[IBIS Ver]   3.2
[File name]   apollo7a.ibs
[File Rev]   0.2
[Date]   Mon Oct 28 12:09:41 CST 2002
[Source]   File originated at Motorola Somerset Design Center.
|   Created by Jim Nissen.
[Notes]   This IBIS model is for the Apollo7 483CBGA ceramic package.
|   The driver and receiver models are characterized up to
|   2.5V mode on the data bus and 2.5V mode on the L3
|   interface. The convention is apollox.ibs, where x
|   is one of the configurations of data bus/L3 bus voltage
|   modes. Following is a table of the code for bus combinations:
|   IBIS model   Bus mode   L3 mode
|   apollo7a.ibs   2.5V   2.5V
|   apollo7b.ibs   2.5V   1.8V
|   apollo7c.ibs   2.5V   1.5V
|   apollo7d.ibs   1.8V   2.5V
|   apollo7e.ibs   1.8V   1.8V
|   apollo7f.ibs   1.8V   1.5V
|   apollo7g.ibs   1.5V   2.5V
|   apollo7h.ibs   1.5V   1.8V
|   apollo7i.ibs   1.5V   1.5V
[Disclaimer]   This information is for modeling purposes only and
|   is not guaranteed.
[Component]   Apollo7
[Manufacturer]  Motorola
[Package]
|   typ   min   max
R_pkg   0.0   0.0   0.0
L_pkg   0.0   0.0   0.0
C_pkg   0.0   0.0   0.0
[Pin]   signal_name   model_name  R_pin   L_pin   C_pin
A2   PLL_CFG0   busio   1E-016   1E-016   1E-016
A3   HRESET_   busio   1E-016   1E-016   1E-016
A4   L3VSEL   rcvr   1E-016   1E-016   1E-016
A5   TT3   busio   1E-016   1E-016   1E-016
A6   A8   busio   1E-016   1E-016   1E-016
A7   A6   busio   1E-016   1E-016   1E-016
A9   DX_   busio   1E-016   1E-016   1E-016
A10   A10   busio   1E-016   1E-016   1E-016
A12   L3_DATAP7   l3io   1E-016   1E-016   1E-016
A13   L3_DATA61   l3io   1E-016   1E-016   1E-016
A14   L3_DATA57   l3io   1E-016   1E-016   1E-016
A15   L3_DATAP6   l3io   1E-016   1E-016   1E-016
A16   L3_DATA53   l3io   1E-016   1E-016   1E-016
A17   L3_DATA52   l3io   1E-016   1E-016   1E-016
A18   L3_DATA48   l3io   1E-016   1E-016   1E-016
A19   L3_DATA47   l3io   1E-016   1E-016   1E-016
A20   L3_DATA44   l3io   1E-016   1E-016   1E-016
A21   L3_DATA41   l3io   1E-016   1E-016   1E-016
A22   GND   POWER   1E-016   1E-016   1E-016
B1   GND   POWER   1E-016   1E-016   1E-016
B2   AVDD   POWER   1E-016   1E-016   1E-016
B3   OVDD   POWER   1E-016   1E-016   1E-016
B4   PMON_OUT_   busio   1E-016   1E-016   1E-016
B5   GND   POWER   1E-016   1E-016   1E-016
B6   OSHD_   busio   1E-016   1E-016   1E-016
B7   TBST_   busio   1E-016   1E-016   1E-016
B8   MCP_   busio   1E-016   1E-016   1E-016
B9   EXT_QUAL   busio   1E-016   1E-016   1E-016
B10   CHKS_   busio   1E-016   1E-016   1E-016
B12   GND   POWER   1E-016   1E-016   1E-016
B13   GVDD   POWER   1E-016   1E-016   1E-016
B14   GND   POWER   1E-016   1E-016   1E-016
B15   GVDD   POWER   1E-016   1E-016   1E-016
B16   GND   POWER   1E-016   1E-016   1E-016
B17   GVDD   POWER   1E-016   1E-016   1E-016
B18   GND   POWER   1E-016   1E-016   1E-016
B19   GVDD   POWER   1E-016   1E-016   1E-016
B20   GND   POWER   1E-016   1E-016   1E-016
B21   GVDD   POWER   1E-016   1E-016   1E-016
B22   L3_DATA39   l3io   1E-016   1E-016   1E-016
C1   TRST_   rcvr   1E-016   1E-016   1E-016
C2   PLL_CFG2   busio   1E-016   1E-016   1E-016
C3   GND   POWER   1E-016   1E-016   1E-016
C4   BMODE1_   busio   1E-016   1E-016   1E-016
C5   OVDD   POWER   1E-016   1E-016   1E-016
C6   BMODE0_   busio   1E-016   1E-016   1E-016
C7   OVDD   POWER   1E-016   1E-016   1E-016
C8   A4   busio   1E-016   1E-016   1E-016
C9   GND   POWER   1E-016   1E-016   1E-016
C10   OVDD   POWER   1E-016   1E-016   1E-016
C12   L3_DATA63   l3io   1E-016   1E-016   1E-016
C13   L3_DATA59   l3io   1E-016   1E-016   1E-016
C14   L3_DATA56   l3io   1E-016   1E-016   1E-016
C15   L3_DATA54   l3io   1E-016   1E-016   1E-016
C16   L3_DATA51   l3io   1E-016   1E-016   1E-016
C17   L3_CLK1   l3io   1E-016   1E-016   1E-016
C18   L3_DATA46   l3io   1E-016   1E-016   1E-016
C19   L3_DATA45   l3io   1E-016   1E-016   1E-016
C20   L3_DATAP4   l3io   1E-016   1E-016   1E-016
C21   GND   POWER   1E-016   1E-016   1E-016
C22   L3_DATA36   l3io   1E-016   1E-016   1E-016
D1   TSIZ2   busio   1E-016   1E-016   1E-016
D2   OVDD   POWER   1E-016   1E-016   1E-016
D4   PLL_CFG3   busio   1E-016   1E-016   1E-016
D6   SYSCLK   rcvr   1E-016   1E-016   1E-016
D7   GND   POWER   1E-016   1E-016   1E-016
D8   SRW0_   busio   1E-016   1E-016   1E-016
D9   A35   busio   1E-016   1E-016   1E-016
D10   A32   busio   1E-016   1E-016   1E-016
D12   GVDD   POWER   1E-016   1E-016   1E-016
D13   GND   POWER   1E-016   1E-016   1E-016
D14   GVDD   POWER   1E-016   1E-016   1E-016
D15   GND   POWER   1E-016   1E-016   1E-016
D16   GVDD   POWER   1E-016   1E-016   1E-016
D17   GND   POWER   1E-016   1E-016   1E-016
D18   GVDD   POWER   1E-016   1E-016   1E-016
D19   GND   POWER   1E-016   1E-016   1E-016
D20   L3_DATA38   l3io   1E-016   1E-016   1E-016
D21   GVDD   POWER   1E-016   1E-016   1E-016
D22   L3_DATA33   l3io   1E-016   1E-016   1E-016
E1   TT4   busio   1E-016   1E-016   1E-016
E2   GND   POWER   1E-016   1E-016   1E-016
E3   OVDD   POWER   1E-016   1E-016   1E-016
E4   TDI   rcvr   1E-016   1E-016   1E-016
E05   GND   POWER   1E-016   1E-016   1E-016
E6   PMON_IN_   busio   1E-016   1E-016   1E-016
E8   A2   busio   1E-016   1E-016   1E-016
E9   OVDD   POWER   1E-016   1E-016   1E-016
E10   A0   busio   1E-016   1E-016   1E-016
E12   L3_DATA62   l3io   1E-016   1E-016   1E-016
E13   L3_DATA58   l3io   1E-016   1E-016   1E-016
E14   L3_ECHO_CLK3   l3io   1E-016   1E-016   1E-016
E15   L3_DATA50   l3io   1E-016   1E-016   1E-016
E16   L3_DATAP5   l3io   1E-016   1E-016   1E-016
E17   L3_DATA43   l3io   1E-016   1E-016   1E-016
E18   L3_ECHO_CLK2   l3io   1E-016   1E-016   1E-016
E19   GVDD   POWER   1E-016   1E-016   1E-016
E20   L3_DATA34   l3io   1E-016   1E-016   1E-016
E21   GND   POWER   1E-016   1E-016   1E-016
E22   L3_ADDR15   l3io   1E-016   1E-016   1E-016
F1   TT0   busio   1E-016   1E-016   1E-016
F2   HPR_   busio   1E-016   1E-016   1E-016
F3   CKSTP_IN_   busio   1E-016   1E-016   1E-016
F4   TT1   busio   1E-016   1E-016   1E-016
F5   OVDD   POWER   1E-016   1E-016   1E-016
F6   LSSD_MODE_   rcvr   1E-016   1E-016   1E-016
F7   PLL_CFG1   busio   1E-016   1E-016   1E-016
F8   WAIT_   busio   1E-016   1E-016   1E-016
F9   SRW1_   busio   1E-016   1E-016   1E-016
F10   GND   POWER   1E-016   1E-016   1E-016
F12   GND   POWER   1E-016   1E-016   1E-016
F13   GVDD   POWER   1E-016   1E-016   1E-016
F14   GND   POWER   1E-016   1E-016   1E-016
F15   GVDD   POWER   1E-016   1E-016   1E-016
F16   GND   POWER   1E-016   1E-016   1E-016
F17   GVDD   POWER   1E-016   1E-016   1E-016
F18   L3_DATA37   l3io   1E-016   1E-016   1E-016
F19   GND   POWER   1E-016   1E-016   1E-016
F20   L3_ADDR17   l3io   1E-016   1E-016   1E-016
F21   GVDD   POWER   1E-016   1E-016   1E-016
F22   L3_ADDR12   l3io   1E-016   1E-016   1E-016
G1   SRESET0_   busio   1E-016   1E-016   1E-016
G3   OVDD   POWER   1E-016   1E-016   1E-016
G4   GND   POWER   1E-016   1E-016   1E-016
G5   AP4   busio   1E-016   1E-016   1E-016
G6   BVSEL   rcvr   1E-016   1E-016   1E-016
G7   GND   POWER   1E-016   1E-016   1E-016
G8   SMI0_   busio   1E-016   1E-016   1E-016
G9   OVDD   POWER   1E-016   1E-016   1E-016
G10   A34   busio   1E-016   1E-016   1E-016
G12   L3_DATA60   l3io   1E-016   1E-016   1E-016
G13   L3_DATA55   l3io   1E-016   1E-016   1E-016
G14   L3_DATA49   l3io   1E-016   1E-016   1E-016
G15   L3_DATA42   l3io   1E-016   1E-016   1E-016
G16   L3_DATA40   l3io   1E-016   1E-016   1E-016
G17   GND   POWER   1E-016   1E-016   1E-016
G18   L3_DATA32   l3io   1E-016   1E-016   1E-016
G19   GVDD   POWER   1E-016   1E-016   1E-016
G20   L3_ADDR13   l3io   1E-016   1E-016   1E-016
G21   GND   POWER   1E-016   1E-016   1E-016
G22   L3_ADDR11   l3io   1E-016   1E-016   1E-016
H1   TDO   busio   1E-016   1E-016   1E-016
H2   AP3   busio   1E-016   1E-016   1E-016
H3   TSIZ1   busio   1E-016   1E-016   1E-016
H4   L1_TSTCLK   rcvr   1E-016   1E-016   1E-016
H5   GND   POWER   1E-016   1E-016   1E-016
H6   IARTRY0_   busio   1E-016   1E-016   1E-016
H7   OVDD   POWER   1E-016   1E-016   1E-016
H8   PLL_CFG4   busio   1E-016   1E-016   1E-016
H10   IARTRY1_   busio   1E-016   1E-016   1E-016
H11   L3_ADDR18   l3io   1E-016   1E-016   1E-016
H12   GVDD   POWER   1E-016   1E-016   1E-016
H13   GND   POWER   1E-016   1E-016   1E-016
H14   GVDD   POWER   1E-016   1E-016   1E-016
H15   GND   POWER   1E-016   1E-016   1E-016
H16   L3_DATA35   l3io   1E-016   1E-016   1E-016
H17   GVDD   POWER   1E-016   1E-016   1E-016
H18   L3_ADDR14   l3io   1E-016   1E-016   1E-016
H19   GND   POWER   1E-016   1E-016   1E-016
H20   L3_ADDR10   l3io   1E-016   1E-016   1E-016
H21   GVDD   POWER   1E-016   1E-016   1E-016
H22   L3_ADDR7   l3io   1E-016   1E-016   1E-016
J1   AP2   busio   1E-016   1E-016   1E-016
J2   L2_TSTCLK   busio   1E-016   1E-016   1E-016
J3   GND   POWER   1E-016   1E-016   1E-016
J4   A33   busio   1E-016   1E-016   1E-016
J5   OVDD   POWER   1E-016   1E-016   1E-016
J6   INT0_   busio   1E-016   1E-016   1E-016
J7   TCK   rcvr   1E-016   1E-016   1E-016
J9   VDD   POWER   1E-016   1E-016   1E-016
J10   GND   POWER   1E-016   1E-016   1E-016
J11   VDD   POWER   1E-016   1E-016   1E-016
J12   GND   POWER   1E-016   1E-016   1E-016
J13   VDD   POWER   1E-016   1E-016   1E-016
J14   GND   POWER   1E-016   1E-016   1E-016
J15   VDD   POWER   1E-016   1E-016   1E-016
J16   L3_ADDR16   l3io   1E-016   1E-016   1E-016
J17   GND   POWER   1E-016   1E-016   1E-016
J18   L3_ADDR8   l3io   1E-016   1E-016   1E-016
J19   GVDD   POWER   1E-016   1E-016   1E-016
J20   L3_ADDR6   l3io   1E-016   1E-016   1E-016
J21   GND   POWER   1E-016   1E-016   1E-016
J22   L3_ADDR5   l3io   1E-016   1E-016   1E-016
K1   BR_   busio   1E-016   1E-016   1E-016
K2   HIT_   busio   1E-016   1E-016   1E-016
K3   OVDD   POWER   1E-016   1E-016   1E-016
K4   TMS   rcvr   1E-016   1E-016   1E-016
K5   GND   POWER   1E-016   1E-016   1E-016
K6   CKSTP_OUT_   busio   1E-016   1E-016   1E-016
K7   QACK_   busio   1E-016   1E-016   1E-016
K8   TT2   busio   1E-016   1E-016   1E-016
K9   GND   POWER   1E-016   1E-016   1E-016
K10   VDD   POWER   1E-016   1E-016   1E-016
K11   GND   POWER   1E-016   1E-016   1E-016
K12   VDD   POWER   1E-016   1E-016   1E-016
K13   GND   POWER   1E-016   1E-016   1E-016
K14   VDD   POWER   1E-016   1E-016   1E-016
K15   GND   POWER   1E-016   1E-016   1E-016
K16   L3_ADDR9   l3io   1E-016   1E-016   1E-016
K17   GVDD   POWER   1E-016   1E-016   1E-016
K18   L3_ADDR4   l3io   1E-016   1E-016   1E-016
K19   GND   POWER   1E-016   1E-016   1E-016
K20   L3_ADDR3   l3io   1E-016   1E-016   1E-016
K21   GVDD   POWER   1E-016   1E-016   1E-016
K22   L3_ADDR1   l3io   1E-016   1E-016   1E-016
L1   TSIZ0   busio   1E-016   1E-016   1E-016
L2   WT_   busio   1E-016   1E-016   1E-016
L3   TBEN   busio   1E-016   1E-016   1E-016
L4   SHD0_   busio   1E-016   1E-016   1E-016
L5   AP0   busio   1E-016   1E-016   1E-016
L6   AP1   busio   1E-016   1E-016   1E-016
L7   OVDD   POWER   1E-016   1E-016   1E-016
L8   SHD1_   busio   1E-016   1E-016   1E-016
L9   VDD   POWER   1E-016   1E-016   1E-016
L10   GND   POWER   1E-016   1E-016   1E-016
L11   VDD   POWER   1E-016   1E-016   1E-016
L12   GND   POWER   1E-016   1E-016   1E-016
L13   VDD   POWER   1E-016   1E-016   1E-016
L14   GND   POWER   1E-016   1E-016   1E-016
L15   VDD   POWER   1E-016   1E-016   1E-016
L16   L3_ADDR2   l3io   1E-016   1E-016   1E-016
L17   GND   POWER   1E-016   1E-016   1E-016
L18   L3_ADDR0   l3io   1E-016   1E-016   1E-016
L19   GVDD   POWER   1E-016   1E-016   1E-016
L20   L3_CNTL0   l3io   1E-016   1E-016   1E-016
L21   GND   POWER   1E-016   1E-016   1E-016
L22   L3_CNTL1   l3io   1E-016   1E-016   1E-016
M1   A9   busio   1E-016   1E-016   1E-016
M2   A7   busio   1E-016   1E-016   1E-016
M3   GND   POWER   1E-016   1E-016   1E-016
M4   GBL_   busio   1E-016   1E-016   1E-016
M5   OVDD   POWER   1E-016   1E-016   1E-016
M6   GND   POWER   1E-016   1E-016   1E-016
M7   A23   busio   1E-016   1E-016   1E-016
M8   A14   busio   1E-016   1E-016   1E-016
M9   GND   POWER   1E-016   1E-016   1E-016
M10   VDD   POWER   1E-016   1E-016   1E-016
M11   GND   POWER   1E-016   1E-016   1E-016
M12   VDD   POWER   1E-016   1E-016   1E-016
M13   GND   POWER   1E-016   1E-016   1E-016
M14   VDD   POWER   1E-016   1E-016   1E-016
M15   L3_DATA31   l3io   1E-016   1E-016   1E-016
M16   L3_DATA20   l3io   1E-016   1E-016   1E-016
M17   GVDD   POWER   1E-016   1E-016   1E-016
M18   L3_DATA21   l3io   1E-016   1E-016   1E-016
M19   GND   POWER   1E-016   1E-016   1E-016
M20   L3_DATA22   l3io   1E-016   1E-016   1E-016
M21   GVDD   POWER   1E-016   1E-016   1E-016
M22   L3_DATA23   l3io   1E-016   1E-016   1E-016
N1   CLK_OUT   busio   1E-016   1E-016   1E-016
N2   A12   busio   1E-016   1E-016   1E-016
N3   OVDD   POWER   1E-016   1E-016   1E-016
N4   A1   busio   1E-016   1E-016   1E-016
N5   A3   busio   1E-016   1E-016   1E-016
N6   A16   busio   1E-016   1E-016   1E-016
N7   A24   busio   1E-016   1E-016   1E-016
N8   TA_   busio   1E-016   1E-016   1E-016
N9   VDD   POWER   1E-016   1E-016   1E-016
N10   GND   POWER   1E-016   1E-016   1E-016
N11   VDD   POWER   1E-016   1E-016   1E-016
N12   GND   POWER   1E-016   1E-016   1E-016
N13   VDD   POWER   1E-016   1E-016   1E-016
N14   GND   POWER   1E-016   1E-016   1E-016
N15   VDD   POWER   1E-016   1E-016   1E-016
N16   L3_DATA18   l3io   1E-016   1E-016   1E-016
N17   GND   POWER   1E-016   1E-016   1E-016
N18   L3_DATA16   l3io   1E-016   1E-016   1E-016
N19   GVDD   POWER   1E-016   1E-016   1E-016
N20   L3_DATA17   l3io   1E-016   1E-016   1E-016
N21   GND   POWER   1E-016   1E-016   1E-016
N22   L3_DATA19   l3io   1E-016   1E-016   1E-016
P1   A20   busio   1E-016   1E-016   1E-016
P2   DTI0   busio   1E-016   1E-016   1E-016
P3   GND   POWER   1E-016   1E-016   1E-016
P4   A21   busio   1E-016   1E-016   1E-016
P5   TS_   busio   1E-016   1E-016   1E-016
P6   DTI3   busio   1E-016   1E-016   1E-016
P7   OVDD   POWER   1E-016   1E-016   1E-016
P8   A13   busio   1E-016   1E-016   1E-016
P9   GND   POWER   1E-016   1E-016   1E-016
P10   VDD   POWER   1E-016   1E-016   1E-016
P11   GND   POWER   1E-016   1E-016   1E-016
P12   VDD   POWER   1E-016   1E-016   1E-016
P13   GND   POWER   1E-016   1E-016   1E-016
P14   VDD   POWER   1E-016   1E-016   1E-016
P15   GND   POWER   1E-016   1E-016   1E-016
P16   L3_DATAP3   l3io   1E-016   1E-016   1E-016
P17   GVDD   POWER   1E-016   1E-016   1E-016
P18   L3_DATA29   l3io   1E-016   1E-016   1E-016
P19   GND   POWER   1E-016   1E-016   1E-016
P20   L3_ECHO_CLK1   l3io   1E-016   1E-016   1E-016
P21   GVDD   POWER   1E-016   1E-016   1E-016
P22   L3_DATAP2   l3io   1E-016   1E-016   1E-016
R1   CI_   busio   1E-016   1E-016   1E-016
R2   A5   busio   1E-016   1E-016   1E-016
R3   BG_   busio   1E-016   1E-016   1E-016
R4   OVDD   POWER   1E-016   1E-016   1E-016
R5   A18   busio   1E-016   1E-016   1E-016
R6   A22   busio   1E-016   1E-016   1E-016
R7   D59   busio   1E-016   1E-016   1E-016
R8   DP4   busio   1E-016   1E-016   1E-016
R9   D60   busio   1E-016   1E-016   1E-016
R10   D28   busio   1E-016   1E-016   1E-016
R11   D23   busio   1E-016   1E-016   1E-016
R12   D17   busio   1E-016   1E-016   1E-016
R13   D50   busio   1E-016   1E-016   1E-016
R14   D2   busio   1E-016   1E-016   1E-016
R15   GVDD   POWER   1E-016   1E-016   1E-016
R16   L3_DATA11   l3io   1E-016   1E-016   1E-016
R17   GND   POWER   1E-016   1E-016   1E-016
R18   L3_DATA24   l3io   1E-016   1E-016   1E-016
R19   GVDD   POWER   1E-016   1E-016   1E-016
R20   L3_DATA28   l3io   1E-016   1E-016   1E-016
R21   GND   POWER   1E-016   1E-016   1E-016
R22   L3_DATA30   l3io   1E-016   1E-016   1E-016
T1   TEA_   busio   1E-016   1E-016   1E-016
T2   ARTRY_   busio   1E-016   1E-016   1E-016
T3   OVDD   POWER   1E-016   1E-016   1E-016
T4   GND   POWER   1E-016   1E-016   1E-016
T5   DTI1   busio   1E-016   1E-016   1E-016
T6   DRDY_   busio   1E-016   1E-016   1E-016
T7   GND   POWER   1E-016   1E-016   1E-016
T8   D33   busio   1E-016   1E-016   1E-016
T9   GND   POWER   1E-016   1E-016   1E-016
T10   D25   busio   1E-016   1E-016   1E-016
T11   D22   busio   1E-016   1E-016   1E-016
T12   D14   busio   1E-016   1E-016   1E-016
T13   GND   POWER   1E-016   1E-016   1E-016
T14   D1   busio   1E-016   1E-016   1E-016
T15   GND   POWER   1E-016   1E-016   1E-016
T16   L3_DATA7   l3io   1E-016   1E-016   1E-016
T17   GVDD   POWER   1E-016   1E-016   1E-016
T18   L3_DATA14   l3io   1E-016   1E-016   1E-016
T19   GND   POWER   1E-016   1E-016   1E-016
T20   L3_DATA25   l3io   1E-016   1E-016   1E-016
T21   GVDD   POWER   1E-016   1E-016   1E-016
T22   L3_DATA27   l3io   1E-016   1E-016   1E-016
U1   AACK_   busio   1E-016   1E-016   1E-016
U2   A11   busio   1E-016   1E-016   1E-016
U3   DTI2   busio   1E-016   1E-016   1E-016
U4   A26   busio   1E-016   1E-016   1E-016
U5   OVDD   POWER   1E-016   1E-016   1E-016
U6   A17   busio   1E-016   1E-016   1E-016
U7   OVDD   POWER   1E-016   1E-016   1E-016
U8   DP6   busio   1E-016   1E-016   1E-016
U9   D31   busio   1E-016   1E-016   1E-016
U10   D29   busio   1E-016   1E-016   1E-016
U11   OVDD   POWER   1E-016   1E-016   1E-016
U12   D10   busio   1E-016   1E-016   1E-016
U13   D13   busio   1E-016   1E-016   1E-016
U14   D5   busio   1E-016   1E-016   1E-016
U15   OVDD   POWER   1E-016   1E-016   1E-016
U16   L3_DATA2   l3io   1E-016   1E-016   1E-016
U17   GND   POWER   1E-016   1E-016   1E-016
U18   L3_DATA9   l3io   1E-016   1E-016   1E-016
U19   GVDD   POWER   1E-016   1E-016   1E-016
U20   L3_DATA15   l3io   1E-016   1E-016   1E-016
U21   GND   POWER   1E-016   1E-016   1E-016
U22   L3_DATA26   l3io   1E-016   1E-016   1E-016
V1   DBG_   busio   1E-016   1E-016   1E-016
V2   GND   POWER   1E-016   1E-016   1E-016
V3   OVDD   POWER   1E-016   1E-016   1E-016
V4   A30   busio   1E-016   1E-016   1E-016
V5   GND   POWER   1E-016   1E-016   1E-016
V6   D56   busio   1E-016   1E-016   1E-016
V7   D32   busio   1E-016   1E-016   1E-016
V8   GND   POWER   1E-016   1E-016   1E-016
V9   OVDD   POWER   1E-016   1E-016   1E-016
V10   D27   busio   1E-016   1E-016   1E-016
V11   D21   busio   1E-016   1E-016   1E-016
V12   GND   POWER   1E-016   1E-016   1E-016
V13   OVDD   POWER   1E-016   1E-016   1E-016
V14   D4   busio   1E-016   1E-016   1E-016
V15   GND   POWER   1E-016   1E-016   1E-016
V16   D53   busio   1E-016   1E-016   1E-016
V17   GVDD   POWER   1E-016   1E-016   1E-016
V18   L3_ECHO_CLK0   l3io   1E-016   1E-016   1E-016
V19   GND   POWER   1E-016   1E-016   1E-016
V20   L3_DATA12   l3io   1E-016   1E-016   1E-016
V21   GVDD   POWER   1E-016   1E-016   1E-016
V22   L3_CLK0   l3io   1E-016   1E-016   1E-016
W1   A28   busio   1E-016   1E-016   1E-016
W2   A27   busio   1E-016   1E-016   1E-016
W3   A29   busio   1E-016   1E-016   1E-016
W4   A15   busio   1E-016   1E-016   1E-016
W5   DP5   busio   1E-016   1E-016   1E-016
W6   D54   busio   1E-016   1E-016   1E-016
W7   GND   POWER   1E-016   1E-016   1E-016
W8   D40   busio   1E-016   1E-016   1E-016
W9   D63   busio   1E-016   1E-016   1E-016
W10   D24   busio   1E-016   1E-016   1E-016
W11   D26   busio   1E-016   1E-016   1E-016
W12   D15   busio   1E-016   1E-016   1E-016
W13   D11   busio   1E-016   1E-016   1E-016
W14   D49   busio   1E-016   1E-016   1E-016
W15   D51   busio   1E-016   1E-016   1E-016
W16   D7   busio   1E-016   1E-016   1E-016
W17   GND   POWER   1E-016   1E-016   1E-016
W18   L3_DATA3   l3io   1E-016   1E-016   1E-016
W19   GVDD   POWER   1E-016   1E-016   1E-016
W20   L3_DATA8   l3io   1E-016   1E-016   1E-016
W21   GND   POWER   1E-016   1E-016   1E-016
W22   L3_DATA13   l3io   1E-016   1E-016   1E-016
Y1   QREQ_   busio   1E-016   1E-016   1E-016
Y2   OVDD   POWER   1E-016   1E-016   1E-016
Y3   GND   POWER   1E-016   1E-016   1E-016
Y4   A19   busio   1E-016   1E-016   1E-016
Y5   OVDD   POWER   1E-016   1E-016   1E-016
Y6   D35   busio   1E-016   1E-016   1E-016
Y7   OVDD   POWER   1E-016   1E-016   1E-016
Y8   D38   busio   1E-016   1E-016   1E-016
Y9   GND   POWER   1E-016   1E-016   1E-016
Y10   OVDD   POWER   1E-016   1E-016   1E-016
Y11   D9   busio   1E-016   1E-016   1E-016
Y12   D20   busio   1E-016   1E-016   1E-016
Y13   GND   POWER   1E-016   1E-016   1E-016
Y14   D12   busio   1E-016   1E-016   1E-016
Y15   GND   POWER   1E-016   1E-016   1E-016
Y16   D47   busio   1E-016   1E-016   1E-016
Y17   OVDD   POWER   1E-016   1E-016   1E-016
Y18   D45   busio   1E-016   1E-016   1E-016
Y19   OVDD   POWER   1E-016   1E-016   1E-016
Y20   GND   POWER   1E-016   1E-016   1E-016
Y21   GVDD   POWER   1E-016   1E-016   1E-016
Y22   L3_DATA10   l3io   1E-016   1E-016   1E-016
AA1   A31   busio   1E-016   1E-016   1E-016
AA2   DP0   busio   1E-016   1E-016   1E-016
AA3   A25   busio   1E-016   1E-016   1E-016
AA4   OVDD   POWER   1E-016   1E-016   1E-016
AA5   GND   POWER   1E-016   1E-016   1E-016
AA6   D37   busio   1E-016   1E-016   1E-016
AA7   D39   busio   1E-016   1E-016   1E-016
AA8   DP3   busio   1E-016   1E-016   1E-016
AA9   D61   busio   1E-016   1E-016   1E-016
AA10   D30   busio   1E-016   1E-016   1E-016
AA11   D8   busio   1E-016   1E-016   1E-016
AA12   D55   busio   1E-016   1E-016   1E-016
AA13   D18   busio   1E-016   1E-016   1E-016
AA14   D52   busio   1E-016   1E-016   1E-016
AA15   OVDD   POWER   1E-016   1E-016   1E-016
AA16   D42   busio   1E-016   1E-016   1E-016
AA17   GND   POWER   1E-016   1E-016   1E-016
AA18   D48   busio   1E-016   1E-016   1E-016
AA19   L3_DATA0   l3io   1E-016   1E-016   1E-016
AA20   L3_DATA4   l3io   1E-016   1E-016   1E-016
AA21   L3_DATA6   l3io   1E-016   1E-016   1E-016
AA22   L3_DATAP1   l3io   1E-016   1E-016   1E-016
AB1   GND   POWER   1E-016   1E-016   1E-016
AB2   DP2   busio   1E-016   1E-016   1E-016
AB3   DP1   busio   1E-016   1E-016   1E-016
AB4   D34   busio   1E-016   1E-016   1E-016
AB5   DP7   busio   1E-016   1E-016   1E-016
AB6   D58   busio   1E-016   1E-016   1E-016
AB7   D36   busio   1E-016   1E-016   1E-016
AB8   D62   busio   1E-016   1E-016   1E-016
AB9   D57   busio   1E-016   1E-016   1E-016
AB10   D41   busio   1E-016   1E-016   1E-016
AB11   D19   busio   1E-016   1E-016   1E-016
AB12   D16   busio   1E-016   1E-016   1E-016
AB13   D3   busio   1E-016   1E-016   1E-016
AB14   D6   busio   1E-016   1E-016   1E-016
AB15   D0   busio   1E-016   1E-016   1E-016
AB16   D43   busio   1E-016   1E-016   1E-016
AB17   D44   busio   1E-016   1E-016   1E-016
AB18   D46   busio   1E-016   1E-016   1E-016
AB19   L3_DATAP0   l3io   1E-016   1E-016   1E-016
AB20   L3_DATA1   l3io   1E-016   1E-016   1E-016
AB21   L3_DATA5   l3io   1E-016   1E-016   1E-016
AB22   GND   POWER   1E-016   1E-016   1E-016
|!!!![Package Model] 'name'  calls name
[Package Model] apollo7_483
[Define Package Model] apollo7_483
[Manufacturer] Motorola Inc.
[OEM] Motorola Inc.
[Description] Apollo7 483 CBGA Package T-Line pkg model
[Number Of Sections] 29
[Number Of Pins]  281
[Pin Numbers]
|Although any length unit can be used for Len, mm is used here.
|signal (1)A(10)
A10   Len=0 L=0.0115888305n /
Len=0 L=0.0115888305n /
Len=0 L=0.0115888305n /
Len=0 L=0.0115888305n /
Len=0 L=0.0115888305n /
Len=13.41889 L=0.40648702n C=0.28033364p R=0.015902141 /
Len=0 L=0.0115888305n /
Len=0 L=0.0115888305n /
Len=0 L=0.0115888305n /
Len=0 L=0.027n /
|signal (2)L3_DATAP(7)
A12   Len=0 L=0.0115888305n /
Len=0 L=0.0115888305n /
Len=0 L=0.0115888305n /
Len=11.64898 L=0.3948527n C=0.28900883p R=0.014814815 /
Len=0 L=0.0115888305n /
Len=3.85077 L=0.3948527n C=0.28900883p R=0.014814815 /
Len=0 L=0.0115888305n /
Len=4.88358 L=0.3948527n C=0.28900883p R=0.014814815 /
Len=0 L=0.0115888305n /
Len=0 L=0.0115888305n /
Len=0 L=0.0115888305n /
Len=0 L=0.0115888305n /
Len=0 L=0.0115888305n /
Len=0 L=0.027n /
|signal (3)L3_DATA(61)
A13   Len=0 L=0.0115888305n /
Len=0 L=0.0115888305n /
Len=0 L=0.0115888305n /
Len=9.55053 L=0.3948527n C=0.28900883p R=0.014814815 /
Len=0 L=0.0115888305n /
Len=0 L=0.0115888305n /
Len=0 L=0.0115888305n /
Len=0 L=0.0115888305n /
Len=0.706 L=0.50999594n C=0.25353685p R=0.017094018 /
Len=0 L=0.0115888305n /
Len=0 L=0.0115888305n /
Len=2.03641 L=0.3948527n C=0.28900883p R=0.014814815 /
Len=0 L=0.0115888305n /
Len=0 L=0.0115888305n /
Len=2.259 L=0.50999594n C=0.25353685p R=0.017094018 /
Len=0 L=0.0115888305n /
Len=0 L=0.0115888305n /
Len=0 L=0.0115888305n /
Len=0 L=0.0115888305n /
Len=5.8358  L=0.3948527n C=0.28900883p R=0.014814815 /
Len=0 L=0.0115888305n /
Len=0 L=0.0115888305n /
Len=0 L=0.0115888305n /
Len=0 L=0.0115888305n /
Len=0 L=0.0115888305n /
Len=0 L=0.027n /
|signal (4)L3_DATA(57)
A14   Len=0 L=0.0115888305n /
Len=0 L=0.0115888305n /
Len=0 L=0.0115888305n /
Len=1.8156348 L=0.3948527n C=0.28900883p R=0.014814815 /
Len=0 L=0.0115888305n /
Len=0 L=0.0115888305n /
Len=0.7243503 L=0.3948527n C=0.28900883p R=0.014814815 /
Len=0 L=0.0115888305n /
Len=0 L=0.0115888305n /
Len=17.844217 L=0.50999594n C=0.25353685p R=0.017094018 /
Len=0 L=0.0115888305n /
Len=0 L=0.027n /
|signal (5)L3_DATAP(6)
A15   Len=0 L=0.0115888305n /
Len=0 L=0.0115888305n /
Len=0 L=0.0115888305n /
Len=12.739074 L=0.41058078n C=0.27740377p R=0.016306954 /
Len=0 L=0.0115888305n /
Len=0 L=0.0115888305n /
Len=3.2260232 L=0.3948527n C=0.28900883p R=0.014814815 /
Len=0 L=0.0115888305n /
Len=0 L=0.0115888305n /
Len=4.40548 L=0.4856581n C=0.26624238p R=0.014814815 /
Len=0 L=0.0115888305n /
Len=0 L=0.027n /
|signal (6)L3_DATA(53)
A16   Len=0 L=0.0115888305n /
Len=0 L=0.0115888305n /
Len=0 L=0.0115888305n /
Len=0 L=0.0115888305n /
Len=0 L=0.0115888305n /
Len=0 L=0.0115888305n /
Len=0 L=0.0115888305n /
Len=20.398748 L=0.49811226n C=0.25958562p R=0.015932914 /
Len=0 L=0.0115888305n /
Len=0 L=0.027n /
|signal (7)L3_DATA(52)
A17   Len=0 L=0.0115888305n /
Len=0 L=0.0115888305n /
Len=0 L=0.0115888305n /
Len=0 L=0.0115888305n /
Len=0 L=0.0115888305n /
Len=12.036658 L=0.42205358n C=0.26950994p R=0.017508417 /
Len=0 L=0.0115888305n /
Len=0 L=0.0115888305n /
Len=8.099174 L=0.4856581n C=0.26624238p R=0.014814815 /
Len=0 L=0.0115888305n /
Len=0 L=0.027n /
|signal (8)L3_DATA(48)
A18   Len=0 L=0.0115888305n /
Len=0 L=0.0115888305n /
Len=0 L=0.0115888305n /
Len=20.387503 L=0.3979373n C=0.2866569p R=0.015094339 /
Len=0 L=0.0115888305n /
Len=0 L=0.0115888305n /
Len=0 L=0.0115888305n /
Len=0 L=0.0115888305n /
Len=0 L=0.0115888305n /
Len=0 L=0.027n /
|signal (9)L3_DATA(47)
A19   Len=0 L=0.0115888305n /
Len=0 L=0.0115888305n /
Len=0 L=0.0115888305n /
Len=6.161309 L=0.3948527n C=0.28900883p R=0.014814815 /
Len=0 L=0.0115888305n /
Len=0 L=0.0115888305n /
Len=7.244859 L=0.3948527n C=0.28900883p R=0.014814815 /
Len=0 L=0.0115888305n /
Len=0 L=0.0115888305n /
Len=6.841765 L=0.51434404n C=0.25139356p R=0.01754386 /
Len=0 L=0.0115888305n /
Len=0 L=0.027n /
|signal (10)PLL_CFG(0)
A2   Len=0 L=0.0115888305n /
Len=0 L=0.0115888305n /
Len=0 L=0.0115888305n /
Len=17.249193 L=0.40563312n C=0.2809526p R=0.015819209 /
Len=0 L=0.0115888305n /
Len=0 L=0.0115888305n /
Len=0 L=0.0115888305n /
Len=0 L=0.0115888305n /
Len=0 L=0.0115888305n /
Len=0 L=0.027n /
|signal (11)L3_DATA(44)
A20   Len=0 L=0.0115888305n /
Len=0 L=0.0115888305n /
Len=0 L=0.0115888305n /
Len=0 L=0.0115888305n /
Len=0 L=0.0115888305n /
Len=9.950993 L=0.40513027n C=0.2813184p R=0.015770609 /
Len=0 L=0.0115888305n /
Len=0 L=0.0115888305n /
Len=10.417507 L=0.4856581n C=0.26624238p R=0.014814815 /
Len=0 L=0.0115888305n /
Len=0 L=0.027n /
|signal (12)L3_DATA(41)
A21   Len=0 L=0.0115888305n /
Len=0 L=0.0115888305n /
Len=0 L=0.0115888305n /
Len=0 L=0.0115888305n /
Len=0 L=0.0115888305n /
Len=10.842759 L=0.3948527n C=0.28900883p R=0.014814815 /
Len=0 L=0.0115888305n /
Len=0 L=0.0115888305n /
Len=9.295238 L=0.51288456n C=0.25210893p R=0.017391305 /
Len=0 L=0.0115888305n /
Len=0 L=0.027n /
|signal (13)HRESET_B
A3   Len=0 L=0.0115888305n /
Len=0 L=0.0115888305n /
Len=0 L=0.0115888305n /
Len=16.309668 L=0.4141186n C=0.27492067p R=0.016666668 /
Len=0 L=0.0115888305n /
Len=0 L=0.0115888305n /
Len=0 L=0.0115888305n /
Len=0 L=0.0115888305n /
Len=0 L=0.0115888305n /
Len=0 L=0.027n /
|signal (14)L3VSEL
A4   Len=0 L=0.0115888305n /
Len=0 L=0.0115888305n /
Len=0 L=0.0115888305n /
Len=9.143236 L=0.40563312n C=0.2809526p R=0.015819209 /
Len=0 L=0.0115888305n /
Len=0 L=0.0115888305n /
Len=0 L=0.0115888305n /
Len=0 L=0.0115888305n /
Len=8.76985 L=0.4856581n C=0.26624238p R=0.014814815 /
Len=0 L=0.0115888305n /
Len=0 L=0.027n /
|signal (15)TT(3)
A5   Len=0 L=0.0115888305n /
Len=0 L=0.0115888305n /
Len=0 L=0.0115888305n /
Len=2.870652 L=0.4309931n C=0.2636639p R=0.018518519 /
Len=0 L=0.0115888305n /
Len=0 L=0.0115888305n /
Len=11.306183 L=0.3948527n C=0.28900883p R=0.014814815 /
Len=0 L=0.0115888305n /
Len=0 L=0.0115888305n /
Len=0 L=0.0115888305n /
Len=0 L=0.027n /
|signal (16)A(8)
A6   Len=0 L=0.0115888305n /
Len=0 L=0.0115888305n /
Len=0 L=0.0115888305n /
Len=0 L=0.0115888305n /
Len=0 L=0.0115888305n /
Len=12.548901 L=0.3948527n C=0.28900883p R=0.014814815 /
Len=0 L=0.0115888305n /
Len=0 L=0.0115888305n /
Len=2.8562863 L=0.49545547n C=0.26097757p R=0.015686275 /
Len=0 L=0.0115888305n /
Len=0 L=0.027n /
|signal (17)A(6)
A7   Len=0 L=0.0115888305n /
Len=0 L=0.0115888305n /
Len=0 L=0.0115888305n /
Len=0 L=0.0115888305n /
Len=0 L=0.0115888305n /
Len=13.991658 L=0.43544444n C=0.26084659p R=0.01904762 /
Len=0 L=0.0115888305n /
Len=0 L=0.0115888305n /
Len=0 L=0.0115888305n /
Len=0 L=0.027n /
|signal (18)DX_B
A9   Len=0 L=0.0115888305n /
Len=0 L=0.0115888305n /
Len=0 L=0.0115888305n /
Len=0 L=0.0115888305n /
Len=0 L=0.0115888305n /
Len=12.404513 L=0.40513027n C=0.2813184p R=0.015770609 /
Len=0 L=0.0115888305n /
Len=0 L=0.0115888305n /
Len=0 L=0.0115888305n /
Len=0 L=0.027n /
|signal (19)A(31)
AA1   Len=0 L=0.0115888305n /
Len=0 L=0.0115888305n /
Len=0 L=0.0115888305n /
Len=0 L=0.0115888305n /
Len=0 L=0.0115888305n /
Len=14.526404 L=0.3948527n C=0.28900883p R=0.014814815 /
Len=0 L=0.0115888305n /
Len=0 L=0.0115888305n /
Len=4.2188034 L=0.4988265n C=0.25921392p R=0.015999999 /
Len=0 L=0.0115888305n /
Len=0 L=0.027n /
|signal (20)D(30)
AA10   Len=0 L=0.0115888305n /
Len=0 L=0.0115888305n /
Len=0 L=0.0115888305n /
Len=10.055819 L=0.4235308n C=0.26852608p R=0.017670684 /
Len=0 L=0.0115888305n /
Len=0 L=0.0115888305n /
Len=0 L=0.0115888305n /
Len=0 L=0.0115888305n /
Len=0 L=0.0115888305n /
Len=0 L=0.027n /
|signal (21)D(8)
AA11   Len=0 L=0.0115888305n /
Len=0 L=0.0115888305n /
Len=0 L=0.0115888305n /
Len=0 L=0.0115888305n /
Len=0 L=0.0115888305n /
Len=12.686109 L=0.4175184n C=0.272576p R=0.017021276 /
Len=0 L=0.0115888305n /
Len=0 L=0.0115888305n /
Len=0 L=0.0115888305n /
Len=0 L=0.027n /
|signal (22)D(55)
AA12   Len=0 L=0.0115888305n /
Len=0 L=0.0115888305n /
Len=0 L=0.0115888305n /
Len=8.9934225 L=0.40648702n C=0.28033364p R=0.015902141 /
Len=0 L=0.0115888305n /
Len=0 L=0.0115888305n /
Len=0 L=0.0115888305n /
Len=0 L=0.0115888305n /
Len=0 L=0.0115888305n /
Len=0 L=0.027n /
|signal (23)D(18)
AA13   Len=0 L=0.0115888305n /
Len=0 L=0.0115888305n /
Len=0 L=0.0115888305n /
Len=0 L=0.0115888305n /
Len=0 L=0.0115888305n /
Len=9.310978 L=0.42298082n C=0.2688915p R=0.017610062 /
Len=0 L=0.0115888305n /
Len=0 L=0.0115888305n /
Len=0 L=0.0115888305n /
Len=0 L=0.027n /
|signal (24)D(52)
AA14   Len=0 L=0.0115888305n /
Len=0 L=0.0115888305n /
Len=0 L=0.0115888305n /
Len=0 L=0.0115888305n /
Len=0 L=0.0115888305n /
Len=9.311807 L=0.4042533n C=0.28195858p R=0.015686275 /
Len=0 L=0.0115888305n /
Len=0 L=0.0115888305n /
Len=0 L=0.0115888305n /
Len=0 L=0.027n /
|signal (25)D(42)
AA16   Len=0 L=0.0115888305n /
Len=0 L=0.0115888305n /
Len=0 L=0.0115888305n /
Len=0 L=0.0115888305n /
Len=0 L=0.0115888305n /
Len=9.206863 L=0.409125n C=0.2784386p R=0.016161617 /
Len=0 L=0.0115888305n /
Len=0 L=0.0115888305n /
Len=0 L=0.0115888305n /
Len=0 L=0.027n /
|signal (26)D(48)
AA18   Len=0 L=0.0115888305n /
Len=0 L=0.0115888305n /
Len=0 L=0.0115888305n /
Len=0 L=0.0115888305n /
Len=0 L=0.0115888305n /
Len=0 L=0.0115888305n /
Len=0 L=0.0115888305n /
Len=16.189888 L=0.4988265n C=0.25921392p R=0.015999999 /
Len=0 L=0.0115888305n /
Len=0 L=0.027n /
|signal (27)L3_DATA(0)
AA19   Len=0 L=0.0115888305n /
Len=0 L=0.0115888305n /
Len=0 L=0.0115888305n /
Len=15.3192425 L=0.4141186n C=0.27492067p R=0.016666668 /
Len=0 L=0.0115888305n /
Len=0 L=0.0115888305n /
Len=0 L=0.0115888305n /
Len=0 L=0.0115888305n /
Len=4.6734977 L=0.4856581n C=0.26624238p R=0.014814815 /
Len=0 L=0.0115888305n /
Len=0 L=0.027n /
|signal (28)DP(0)
AA2   Len=0 L=0.0115888305n /
Len=0 L=0.0115888305n /
Len=0 L=0.0115888305n /
Len=13.9443 L=0.4175184n C=0.272576p R=0.017021276 /
Len=0 L=0.0115888305n /
Len=0 L=0.0115888305n /
Len=0 L=0.0115888305n /
Len=0 L=0.0115888305n /
Len=0 L=0.0115888305n /
Len=0 L=0.027n /
|signal (29)L3_DATA(4)
AA20   Len=0 L=0.0115888305n /
Len=0 L=0.0115888305n /
Len=0 L=0.0115888305n /
Len=20.089561 L=0.4005851n C=0.2846683p R=0.015339232 /
Len=0 L=0.0115888305n /
Len=0 L=0.0115888305n /
Len=0 L=0.0115888305n /
Len=0 L=0.0115888305n /
Len=0 L=0.0115888305n /
Len=0 L=0.027n /
|signal (30)L3_DATA(6)
AA21   Len=0 L=0.0115888305n /
Len=0 L=0.0115888305n /
Len=0 L=0.0115888305n /
Len=12.642385 L=0.40563312n C=0.2809526p R=0.015819209 /
Len=0 L=0.0115888305n /
Len=0 L=0.0115888305n /
Len=5.5898447 L=0.3948527n C=0.28900883p R=0.014814815 /
Len=0 L=0.0115888305n /
Len=0 L=0.0115888305n /
Len=2.045 L=0.4856581n C=0.26624238p R=0.014814815 /
Len=0 L=0.0115888305n /
Len=0 L=0.027n /
|signal (31)L3_DATAP(1)
AA22   Len=0 L=0.0115888305n /
Len=0 L=0.0115888305n /
Len=0 L=0.0115888305n /
Len=0 L=0.0115888305n /
Len=0 L=0.0115888305n /
Len=19.885822 L=0.41508406n C=0.27425075p R=0.016766466 /
Len=0 L=0.0115888305n /
Len=0 L=0.0115888305n /
Len=0 L=0.0115888305n /
Len=0 L=0.027n /
|signal (32)A(25)
AA3   Len=0 L=0.0115888305n /
Len=0 L=0.0115888305n /
Len=0 L=0.0115888305n /
Len=6.230401 L=0.41124985n C=0.27693075p R=0.016374268 /
Len=0 L=0.0115888305n /
Len=0 L=0.0115888305n /
Len=10.2146435 L=0.3948527n C=0.28900883p R=0.014814815 /
Len=0 L=0.0115888305n /
Len=0 L=0.0115888305n /
Len=0 L=0.0115888305n /
Len=0 L=0.027n /
|signal (33)D(37)
AA6   Len=0 L=0.0115888305n /
Len=0 L=0.0115888305n /
Len=0 L=0.0115888305n /
Len=12.79767 L=0.4244969n C=0.26788652p R=0.017777778 /
Len=0 L=0.0115888305n /
Len=0 L=0.0115888305n /
Len=0 L=0.0115888305n /
Len=0 L=0.0115888305n /
Len=0 L=0.0115888305n /
Len=0 L=0.027n /
|signal (34)D(39)
AA7   Len=0 L=0.0115888305n /
Len=0 L=0.0115888305n /
Len=0 L=0.0115888305n /
Len=8.458708 L=0.4284607n C=0.26529408p R=0.018225418 /
Len=0 L=0.0115888305n /
Len=0 L=0.0115888305n /
Len=2.8026388 L=0.3948527n C=0.28900883p R=0.014814815 /
Len=0 L=0.0115888305n /
Len=0 L=0.0115888305n /
Len=0 L=0.0115888305n /
Len=0 L=0.027n /
|signal (35)DP(3)
AA8   Len=0 L=0.0115888305n /
Len=0 L=0.0115888305n /
Len=0 L=0.0115888305n /
Len=0 L=0.0115888305n /
Len=0 L=0.0115888305n /
Len=12.295625 L=0.41702917n C=0.27291092p R=0.016969698 /
Len=0 L=0.0115888305n /
Len=0 L=0.0115888305n /
Len=0 L=0.0115888305n /
Len=0 L=0.027n /
|signal (36)D(61)
AA9   Len=0 L=0.0115888305n /
Len=0 L=0.0115888305n /
Len=0 L=0.0115888305n /
Len=9.541427 L=0.40351424n C=0.28250036p R=0.015615616 /
Len=0 L=0.0115888305n /
Len=0 L=0.0115888305n /
Len=0 L=0.0115888305n /
Len=0 L=0.0115888305n /
Len=0 L=0.0115888305n /
Len=0 L=0.027n /
|signal (37)D(41)
AB10   Len=0 L=0.0115888305n /
Len=0 L=0.0115888305n /
Len=0 L=0.0115888305n /
Len=9.982628 L=0.4216125n C=0.26980507p R=0.017460316 /
Len=0 L=0.0115888305n /
Len=0 L=0.0115888305n /
Len=0 L=0.0115888305n /
Len=0 L=0.0115888305n /
Len=5.1796894 L=0.4856581n C=0.26624238p R=0.014814815 /
Len=0 L=0.0115888305n /
Len=0 L=0.027n /
|signal (38)D(19)
AB11   Len=0 L=0.0115888305n /
Len=0 L=0.0115888305n /
Len=0 L=0.0115888305n /
Len=5.428834 L=0.4305046n C=0.2639768p R=0.018461538 /
Len=0 L=0.0115888305n /
Len=0 L=0.0115888305n /
Len=5.922026 L=0.3948527n C=0.28900883p R=0.014814815 /
Len=0 L=0.0115888305n /
Len=0 L=0.0115888305n /
Len=0 L=0.0115888305n /
Len=0 L=0.027n /
|signal (39)D(16)
AB12   Len=0 L=0.0115888305n /
Len=0 L=0.0115888305n /
Len=0 L=0.0115888305n /
Len=9.974475 L=0.40513027n C=0.2813184p R=0.015770609 /
Len=0 L=0.0115888305n /
Len=0 L=0.0115888305n /
Len=0 L=0.0115888305n /
Len=0 L=0.0115888305n /
Len=0 L=0.0115888305n /
Len=0 L=0.027n /
|signal (40)D(3)
AB13   Len=0 L=0.0115888305n /
Len=0 L=0.0115888305n /
Len=0 L=0.0115888305n /
Len=12.418953 L=0.43295923n C=0.26241204p R=0.018749999 /
Len=0 L=0.0115888305n /
Len=0 L=0.0115888305n /
Len=0 L=0.0115888305n /
Len=0 L=0.0115888305n /
Len=0 L=0.0115888305n /
Len=0 L=0.027n /
|signal (41)D(6)
AB14   Len=0 L=0.0115888305n /
Len=0 L=0.0115888305n /
Len=0 L=0.0115888305n /
Len=9.859826 L=0.3982201n C=0.28644314p R=0.015120275 /
Len=0 L=0.0115888305n /
Len=0 L=0.0115888305n /
Len=0 L=0.0115888305n /
Len=0 L=0.0115888305n /
Len=0 L=0.0115888305n /
Len=0 L=0.027n /
|signal (42)D(0)
AB15   Len=0 L=0.0115888305n /
Len=0 L=0.0115888305n /
Len=0 L=0.0115888305n /
Len=10.167481 L=0.4384681n C=0.25896695p R=0.019417476 /
Len=0 L=0.0115888305n /
Len=0 L=0.0115888305n /
Len=0 L=0.0115888305n /
Len=0 L=0.0115888305n /
Len=0 L=0.0115888305n /
Len=0 L=0.027n /
|signal (43)D(43)
AB16   Len=0 L=0.0115888305n /
Len=0 L=0.0115888305n /
Len=0 L=0.0115888305n /
Len=0 L=0.0115888305n /
Len=0 L=0.0115888305n /
Len=0 L=0.0115888305n /
Len=0 L=0.0115888305n /
Len=10.701811 L=0.50999594n C=0.25353685p R=0.017094018 /
Len=0 L=0.0115888305n /
Len=0 L=0.027n /
|signal (44)D(44)
AB17   Len=0 L=0.0115888305n /
Len=0 L=0.0115888305n /
Len=0 L=0.0115888305n /
Len=0 L=0.0115888305n /
Len=0 L=0.0115888305n /
Len=0 L=0.0115888305n /
Len=0 L=0.0115888305n /
Len=10.432901 L=0.5015632n C=0.25779957p R=0.016260162 /
Len=0 L=0.0115888305n /
Len=0 L=0.027n /
|signal (45)D(46)
AB18   Len=0 L=0.0115888305n /
Len=0 L=0.0115888305n /
Len=0 L=0.0115888305n /
Len=0 L=0.0115888305n /
Len=0 L=0.0115888305n /
Len=0 L=0.0115888305n /
Len=0 L=0.0115888305n /
Len=12.491081 L=0.50877017n C=0.2541477p R=0.016969698 /
Len=0 L=0.0115888305n /
Len=0 L=0.027n /
|signal (46)L3_DATAP(0)
AB19   Len=0 L=0.0115888305n /
Len=0 L=0.0115888305n /
Len=0 L=0.0115888305n /
Len=20.269188 L=0.4005851n C=0.2846683p R=0.015339232 /
Len=0 L=0.0115888305n /
Len=0 L=0.0115888305n /
Len=0 L=0.0115888305n /
Len=0 L=0.0115888305n /
Len=0 L=0.0115888305n /
Len=0 L=0.027n /
|signal (47)DP(2)
AB2   Len=0 L=0.0115888305n /
Len=0 L=0.0115888305n /
Len=0 L=0.0115888305n /
Len=18.220663 L=0.42589125n C=0.26696882p R=0.017933724 /
Len=0 L=0.0115888305n /
Len=0 L=0.0115888305n /
Len=0 L=0.0115888305n /
Len=0 L=0.0115888305n /
Len=0 L=0.0115888305n /
Len=0 L=0.027n /
|signal (48)L3_DATA(1)
AB20   Len=0 L=0.0115888305n /
Len=0 L=0.0115888305n /
Len=0 L=0.0115888305n /
Len=5.763905 L=0.3948527n C=0.28900883p R=0.014814815 /
Len=0 L=0.0115888305n /
Len=0 L=0.0115888305n /
Len=14.503824 L=0.41596586n C=0.27364174p R=0.016858237 /
Len=0 L=0.0115888305n /
Len=0 L=0.0115888305n /
Len=0 L=0.0115888305n /
Len=0 L=0.027n /
|signal (49)L3_DATA(5)
AB21   Len=0 L=0.0115888305n /
Len=0 L=0.0115888305n /
Len=0 L=0.0115888305n /
Len=9.798785 L=0.4042533n C=0.28195858p R=0.015686275 /
Len=0 L=0.0115888305n /
Len=0 L=0.0115888305n /
Len=5.6927915 L=0.3948527n C=0.28900883p R=0.014814815 /
Len=0 L=0.0115888305n /
Len=0 L=0.0115888305n /
Len=4.403771 L=0.4856581n C=0.26624238p R=0.014814815 /
Len=0 L=0.0115888305n /
Len=0 L=0.027n /
|signal (50)DP(1)
AB3   Len=0 L=0.0115888305n /
Len=0 L=0.0115888305n /
Len=0 L=0.0115888305n /
Len=0 L=0.0115888305n /
Len=0 L=0.0115888305n /
Len=15.091909 L=0.41884163n C=0.27167422p R=0.017161716 /
Len=0 L=0.0115888305n /
Len=0 L=0.0115888305n /
Len=0 L=0.0115888305n /
Len=0 L=0.027n /
|signal (51)D(34)
AB4   Len=0 L=0.0115888305n /
Len=0 L=0.0115888305n /
Len=0 L=0.0115888305n /
Len=0 L=0.0115888305n /
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[End Package Model]
| Models and submodels in the file (3): busio (I/O), rcvr (Input), l3io (I/O)
